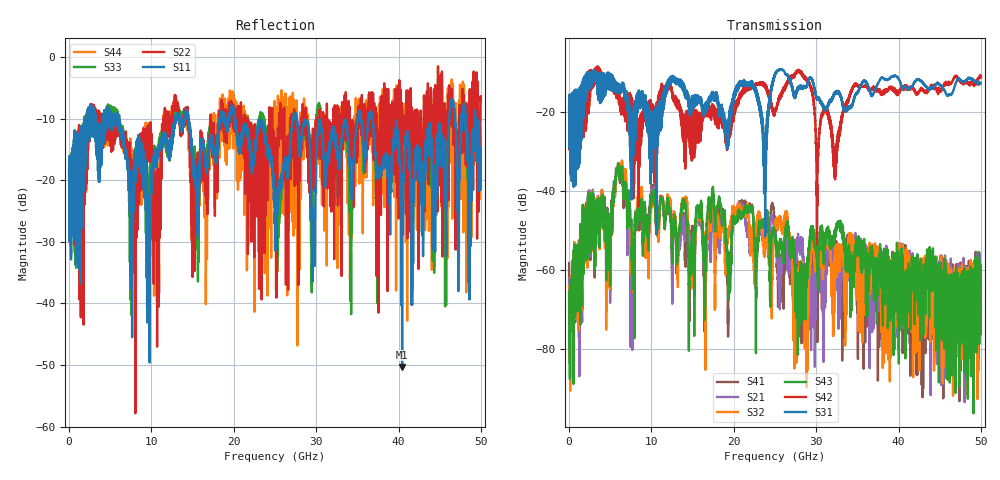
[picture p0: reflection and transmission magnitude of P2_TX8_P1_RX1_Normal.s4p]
!Keysight Technologies,N5225B,MY57041031,A.13.20.10
!Date: Friday, May 31, 2019 11:15:16
!Correction: S11(Full 4 Port(1,2,3,4))
!S12(Full 4 Port(1,2,3,4))
!S13(Full 4 Port(1,2,3,4))
!S14(Full 4 Port(1,2,3,4))
!S21(Full 4 Port(1,2,3,4))
!S22(Full 4 Port(1,2,3,4))
!S23(Full 4 Port(1,2,3,4))
!S24(Full 4 Port(1,2,3,4))
!S31(Full 4 Port(1,2,3,4))
!S32(Full 4 Port(1,2,3,4))
!S33(Full 4 Port(1,2,3,4))
!S34(Full 4 Port(1,2,3,4))
!S41(Full 4 Port(1,2,3,4))
!S42(Full 4 Port(1,2,3,4))
!S43(Full 4 Port(1,2,3,4))
!S44(Full 4 Port(1,2,3,4))
!S4P File: Measurements: <S11,S12,S13,S14>,
!<S21,S22,S23,S24>,
!<S31,S32,S33,S34>,
!<S41,S42,S43,S44>:
# Hz S  dB  R 50.0
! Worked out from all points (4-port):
!   5000 points, 10 MHz to 50 GHz, reference 50 ohm
!   strongest paths, dB at 10 MHz, 12.51 GHz, 25.01 GHz, 37.51 GHz, 50 GHz:
!     S31: -19.3, -11.6, -10.3, -12.8, -12.8
!     S42: -19.5, -14.8, -19.7, -14.5, -11.3
!     S43: -65.7, -56.6, -51.0, -59.8, -63.9
!     S32: -64.1, -51.3, -48.4, -54.6, -65.2
!     S21: -62.1, -59.6, -51.5, -61.0, -58.6
!     S41: -58.2, -62.6, -48.4, -65.3, -69.7
!   lowest |S11| = -50.3 dB at 40.44 GHz (marker M1), VSWR 1.01, Z = 49.8 - j0.178 ohm
!   |S11| at or under -10 dB: 20.17 GHz to 27.18 GHz (7.013 GHz wide, 29.6 % of centre); 27.67 GHz to 35.04 GHz (7.369 GHz wide, 23.5 % of centre); 36.79 GHz to 46.17 GHz (9.379 GHz wide, 22.6 % of centre)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
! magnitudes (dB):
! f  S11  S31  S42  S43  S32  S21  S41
! 10 MHz  -19.7  -19.3  -19.5  -65.7  -64.1  -62.1  -58.2
! 6.3 GHz  -13.0  -14.9  -18.7  -34.4  -32.9  -33.4  -35.1
! 7.68 GHz  -24.6  -21.3  -18.9  -52.0  -56.1  -64.9  -52.3
! 10.14 GHz  -18.7  -26.1  -19.7  -42.6  -43.6  -41.0  -39.9
! 27.49 GHz  -9.4  -15.5  -10.3  -70.5  -70.7  -54.8  -56.8
! 40.44 GHz  -50.3  -14.2  -13.8  -68.0  -60.9  -63.4  -54.8
! 50 GHz  -15.1  -12.8  -11.3  -63.9  -65.2  -58.6  -69.7
